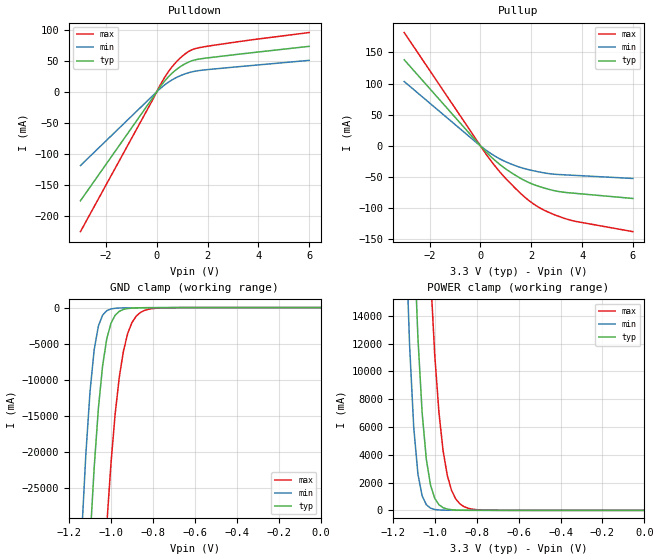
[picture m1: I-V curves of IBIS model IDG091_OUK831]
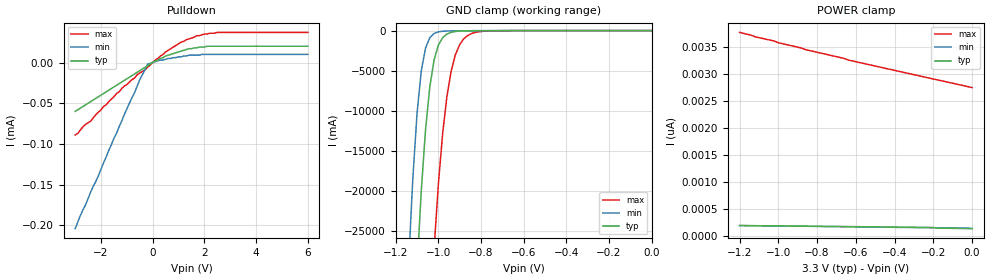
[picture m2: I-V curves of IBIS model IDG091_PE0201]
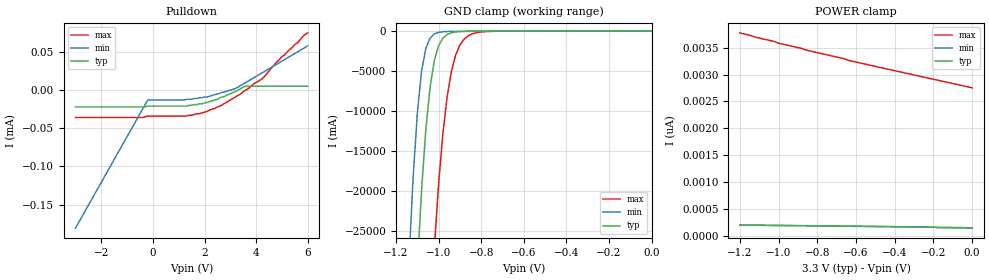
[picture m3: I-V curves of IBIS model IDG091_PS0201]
[IBIS Ver]   2.1
[File name]   dac5686.ibs
[File Rev]   1.0
[Date]   20 Oct 2004
[Source]   Preliminary Model
[Notes]
   Technology type GS30
[Disclaimer]   Please be aware that in the absence of a written agreement
|   Texas Instruments(TI) assumes no liability for:
|   (1) The accuracy of the IBIS models provided to your company
|   (2) The proper functioning of these Models in your design
|   or for any resulting applications;or
|   property rights resulting from your use of these models.
|   TI provides IBIS Models as a service to our customers and
|   therefore reserves the right to limit distribution of the
|   Models.
[Copyright]   Property of Texas Instruments Incorporated.
|   Unauthorised reproduction and/or distribution is strictly.
|   prohibited.
|   This product is protected under copyright law and trade
|   secret law as an unpublished work.
|   Created 1999,(C) Copyright 1999-2001,
|   Texas Instruments Incorporated., All Rights Reserved.
|   These commodities are under the U.S.
|   Government distribution license control.As such,they are not
|   to be re-exported without the prior approval of the U.S.
|   Department of Commerce.
[Component]   DAC5686
[Manufacturer]   Texas Instruments
[Package]
|   typ   min   max
R_pkg   0.055   0.003   0.074
L_pkg   3.746nH   2.468nH   4.445nH
C_pkg   0.413pF   0.342pF   0.498pF
[Pin]   signal_name   model_name   R_pin   L_pin   C_pin
   1   AGND   GND   0.057   4.338nH   0.438pF
   2   AVDD   POWER   0.058   4.085nH   0.472pF
   3   AVDD   POWER   0.060   4.040nH   0.456pF
   4   AGND   GND   0.060   4.008nH   0.448pF
   5   IOUTB1   NC   0.063   4.018nH   0.444pF
   6   IOUTB2   NC   0.063   3.971nH   0.427pF
   7   AGND   GND   0.063   3.935nH   0.421pF
   8   AVDD   POWER   0.064   3.883nH   0.415pF
   9   AGND   GND   0.065   3.824nH   0.403pF
   10   AVDD   POWER   0.068   3.805nH   0.392pF
   11   EXTIO   NC   0.068   3.786nH   0.384pF
   12   AGND   GND   0.069   3.777nH   0.394pF
   13   BIASJ   NC   0.067   3.733nH   0.405pF
   14   AVDD   POWER   0.069   3.778nH   0.392pF
   15   EXTLO   NC   0.065   3.785nH   0.385pF
   16   AVDD   POWER   0.065   3.827nH   0.394pF
   17   AGND   GND   0.063   3.848nH   0.403pF
   18   AVDD   POWER   0.065   3.921nH   0.416pF
   19   AGND   GND   0.062   3.955nH   0.419pF
   20   IOUTA2   NC   0.062   3.910nH   0.417pF
   21   IOUTA1   NC   0.061   3.964nH   0.439pF
   22   AGND   GND   0.060   3.962nH   0.451pF
   23   AVDD   POWER   0.057   4.045nH   0.463pF
   24   AVDD   POWER   0.003   2.474nH   0.389pF
   25   AGND   GND   0.003   2.545nH   0.342pF
   26   DVDD   POWER   0.046   3.901nH   0.416pF
   27   DGND   GND   0.046   3.704nH   0.454pF
   28   SDENB   IDG091_PE0201   0.049   3.801nH   0.445pF
   29   SCLK   IDG091_PE0201   0.049   3.745nH   0.435pF
   30   SDIO   IDG091_OUK831   0.050   3.712nH   0.426pF
   31   SDO   OUK831   0.051   3.586nH   0.402pF
   32   DVDD   POWER   0.054   3.629nH   0.402pF
   33   TXENABLE   IDG091_PE0201   0.056   3.632nH   0.401pF
   34   DA15   IDG091_PE0201   0.057   3.603nH   0.391pF
   35   DA14   IDG091_PE0201   0.057   3.584nH   0.382pF
   36   DA13   IDG091_PE0201   0.060   3.589nH   0.375pF
   37   DVDD   POWER   0.055   3.476nH   0.377pF
   38   DGND   GND   0.054   3.575nH   0.368pF
   39   DA12   IDG091_PE0201   0.052   3.487nH   0.374pF
   40   DA11   IDG091_PE0201   0.049   3.490nH   0.369pF
   41   DA10   IDG091_PE0201   0.051   3.608nH   0.383pF
   42   DA9   IDG091_PE0201   0.049   3.610nH   0.391pF
   43   DA8   IDG091_PE0201   0.049   3.739nH   0.409pF
   44   DVDD   POWER   0.050   3.767nH   0.410pF
   45   DGND   GND   0.045   3.716nH   0.410pF
   46   IOVDD   POWER   0.048   3.837nH   0.434pF
   47   IOGND   GND   0.041   3.703nH   0.440pF
   48   DA7   IDG091_PE0201   0.043   3.923nH   0.456pF
   49   DA6   IDG091_PE0201   0.003   2.468nH   0.385pF
   50   DA5   IDG091_PE0201   0.003   2.537nH   0.345pF
   51   DA4   IDG091_PE0201   0.057   4.445nH   0.457pF
   52   DA3   IDG091_PE0201   0.059   4.279nH   0.498pF
   53   DA2   IDG091_PE0201   0.062   4.315nH   0.477pF
   54   DA1   IDG091_PE0201   0.062   4.283nH   0.469pF
   55   DA0   IDG091_PE0201   0.065   4.328nH   0.468pF
   56   DVDD   POWER   0.066   4.202nH   0.444pF
   57   DGND   GND   0.066   4.126nH   0.434pF
   58   CLKGND   GND   0.065   4.106nH   0.433pF
   59   CLK1   IOH121   0.067   4.025nH   0.419pF
   60   CLK1C   IOH121   0.071   4.030nH   0.410pF
   61   CLKVDD   POWER   0.069   3.947nH   0.398pF
   62   CLK2   IOH121   0.070   3.905nH   0.405pF
   63   CLK2C   IOH121   0.073   3.898nH   0.417pF
   64   CLKGND   GND   0.074   3.911nH   0.399pF
   65   PLLGND   GND   0.073   3.916nH   0.390pF
   66   LPF   IOH121   0.073   3.956nH   0.401pF
   67   PLLVDD   POWER   0.073   3.992nH   0.410pF
   68   DVDD   POWER   0.073   4.041nH   0.421pF
   69   DGND   GND   0.070   4.042nH   0.425pF
   70   PLLLOCK   OUK831   0.069   4.043nH   0.427pF
   71   DB0   IDG091_PE0201   0.067   4.067nH   0.443pF
   72   DB1   IDG091_PE0201   0.064   4.039nH   0.448pF
   73   DB2   IDG091_PE0201   0.063   4.015nH   0.459pF
   74   DB3   IDG091_PE0201   0.060   4.174nH   0.485pF
   75   DB4   IDG091_PE0201   0.003   2.539nH   0.348pF
   76   DB5   IDG091_PE0201   0.049   3.991nH   0.426pF
   77   DB6   IDG091_PE0201   0.049   3.840nH   0.463pF
   78   DB7   IDG091_PE0201   0.050   3.788nH   0.443pF
   79   IOGND   GND   0.049   3.757nH   0.435pF
   80   IOVDD   POWER   0.051   3.777nH   0.431pF
   81   DGND   GND   0.052   3.658nH   0.407pF
   82   DVDD   POWER   0.052   3.650nH   0.403pF
   83   DB8   IDG091_PE0201   0.055   3.650nH   0.400pF
   84   DB9   IDG091_PE0201   0.055   3.597nH   0.390pF
   85   DB10   IDG091_PE0201   0.056   3.550nH   0.378pF
   86   DB11   IDG091_PE0201   0.057   3.532nH   0.370pF
   87   DB12   IDG091_PE0201   0.054   3.428nH   0.372pF
   88   DGND   GND   0.058   3.631nH   0.370pF
   89   DVDD   POWER   0.055   3.479nH   0.373pF
   90   DB13   IDG091_PE0201   0.056   3.531nH   0.369pF
   91   DB14   IDG091_PE0201   0.057   3.597nH   0.380pF
   92   DB15   IDG091_PE0201   0.056   3.611nH   0.388pF
   93   DGND   GND   0.055   3.678nH   0.403pF
   94   PHSTR   IDG091_PE0201   0.054   3.732nH   0.407pF
   95   RESETB   IDG091_PS0201   0.049   3.619nH   0.402pF
   96   SLEEP   IDG091_PE0201   0.051   3.713nH   0.425pF
   97   TESTMODE   IDG091_PE0201   0.047   3.658nH   0.433pF
   98   QFLAG   IDG091_PE0201   0.050   3.841nH   0.452pF
   99   DGND   GND   0.003   2.476nH   0.392pF
  100   DVDD   POWER   0.003   2.547nH   0.344pF
| Models and submodels in the file (5): IDG091_OUK831 (I/O), IDG091_PE0201 (Input), IDG091_PS0201 (Input), OUK831 (3-state), IOH121 (Input)
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[Model]   IDG091_OUK831
Model_type   I/O
Enable   Active-Low
Polarity   Non-Inverting
| signals   A, GZ, Y
Vinl = 0.8V
Vinh = 2.0V
Vmeas = 1.5
|   typ   min   max
C_comp   3.5921p   3.4389p   4.1227p
|   typ   min   max
[Temperature Range]   25   -40.0   125
|   typ   min   max
[Voltage Range]   3.30V   3.00V   3.60V
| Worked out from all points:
|   slope of the pulldown table from 0 to 0.495 V, typ, clamps not added: 19.3 ohm
|   slope of the pullup table from 0 to 0.495 V, typ, clamps not added: 24.2 ohm
|   GND clamp passes 1 mA (typ) near -0.58 V on its own axis
|   POWER clamp passes 1 mA (typ) near -0.64 V on its own axis
[Pulldown]
|   Voltage   I(typ)   I(min)   I(max)
-3V       -175.9mA   -119.1mA   -225.8mA
-200mV    -12.18mA   -7.956mA   -16.01mA
200mV     11.61mA    7.405mA    15.55mA
400mV     21.52mA    13.77mA    28.85mA
600mV     29.89mA    19.16mA    40.1mA
1V        42.47mA    27.25mA    57.28mA
1.3V      48.84mA    31.34mA    66.22mA
1.7V      53.08mA    34.51mA    71.52mA
3.6V      62.5mA     41.98mA    83.19mA
6V        73.47mA    50.83mA    95.74mA
[GND_clamp]
|   Voltage   I(typ)   I(min)   I(max)
-1.2V     -102.7A    -74.41A    -154.1A
-1.14V    -57.55A    -31.62A    -106.7A
-1.1V     -32.35A    -11.69A    -77.65A
-1.08V    -22.13A    -5.816A    -64.19A
-1.06V    -13.97A    -2.559A    -51.65A
-1.04V    -8.085A    -1.052A    -40.23A
-1.02V    -4.316A    -431.8mA   -30.14A
-980mV    -1.059A    -97.69mA   -14.73A
-960mV    -513.4mA   -60.94mA   -9.568A
-920mV    -131.1mA   -37.25mA   -3.566A
-880mV    -45.19mA   -28.49mA   -1.203A
0V        -130.5pA   -109.2pA   -2.072nA
[Pullup]
|   Voltage   I(typ)   I(min)   I(max)
-3V       138.1mA    103.2mA    181.7mA
-200mV    9.146mA    6.727mA    12.21mA
300mV     -12.88mA   -9.22mA    -17.63mA
900mV     -34.12mA   -23.64mA   -48.03mA
1.7V      -54.7mA    -36.06mA   -80.58mA
2.1V      -62.01mA   -39.98mA   -93.36mA
2.4V      -66.16mA   -42.43mA   -100.8mA
2.9V      -71.73mA   -45.34mA   -110.1mA
3.3V      -74.37mA   -46.38mA   -116.1mA
3.8V      -76.3mA    -47.46mA   -121.4mA
6V        -84.26mA   -52.21mA   -137.4mA
[POWER_clamp]
|   Voltage   I(typ)   I(min)   I(max)
-1.2V     83.43A     59.64A     127.8A
-1.14V    41.42A     20.8A      82.7A
-1.12V    29.85A     11.95A     68.94A
-1.1V     20.06A     5.958A     56.04A
-1.08V    12.41A     2.607A     44.19A
-1.06V    7.027A     1.048A     33.6A
-1.04V    3.679A     406.1mA    24.47A
-1.02V    1.819A     157.9mA    16.99A
-960mV    192.4mA    15.59mA    4.285A
-920mV    44.41mA    7.991mA    1.453A
-880mV    12.4mA     6.125mA    468.3mA
0V        154.5pA    161.2pA    3.029nA
[Ramp]
|   I(typ)   I(min)   I(max)
dV/dt_r   1.267/1.474n   0.957/2.769n   1.564/0.824n
dV/dt_f   1.332/1.513n   0.961/2.653n   1.616/0.826n
[Model]   IDG091_PE0201
Model_type   Input
Polarity   Non-Inverting
| signals   A, Y
Vinl = 0.8V
Vinh = 2.0V
|   typ   min   max
C_comp   3.016p   2.9215p   3.4873p
|   typ   min   max
[Temperature Range]   25   -40.0   125
|   typ   min   max
[Voltage Range]   3.30V   3.00V   3.60V
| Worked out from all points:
|   slope of the pulldown table from 0 to 0.495 V, typ, clamps not added: 62.7 kohm
|   GND clamp passes 1 mA (typ) near -0.58 V on its own axis
[Pulldown]
|   Voltage   I(typ)   I(min)   I(max)
-3V       -60uA      -204uA     -89uA
-2.6V     -52uA      -175uA     -76uA
-2.4V     -48uA      -159uA     -72uA
-2.1V     -42uA      -139uA     -61uA
-1.1V     -22uA      -64uA      -29uA
-500mV    -10uA      -21uA      -13uA
-200mV    -4uA       -2uA       -6uA
500mV     8uA        4uA        13uA
1.1V      14uA       7uA        25uA
1.7V      18uA       9uA        33uA
2.5V      20uA       10uA       37uA
6V        20uA       10uA       37uA
[GND_clamp]
|   Voltage   I(typ)   I(min)   I(max)
-1.2V     -98.78A    -71.42A    -148.8A
-1.14V    -54.21A    -29.33A    -101.8A
-1.1V     -29.69A    -10.34A    -73.18A
-1.08V    -19.94A    -5.01A     -60A
-1.06V    -12.33A    -2.162A    -47.8A
-1.04V    -6.983A    -880.6mA   -36.79A
-1.02V    -3.664A    -361.6mA   -27.18A
-980mV    -884.2mA   -83.74mA   -12.87A
-960mV    -428mA     -53.16mA   -8.232A
-920mV    -110.2mA   -33.2mA    -3A
-880mV    -38.87mA   -25.56mA   -1.002A
0V        -427.6fA   -2.728fA   -107pA
[POWER_clamp]
|   Voltage   I(typ)   I(min)   I(max)
-1.2V     197.2pA    197.2pA    3.775nA
-1.14V    194.5pA    194.5pA    3.723nA
-1.12V    194.5pA    193.6pA    3.695nA
-1.02V    191pA      190.1pA    3.613nA
-1V       191pA      189.2pA    3.583nA
-880mV    187.4pA    184.7pA    3.485nA
-860mV    187.4pA    184.7pA    3.456nA
-660mV    178.5pA    175.9pA    3.293nA
-640mV    178.1pA    175pA      3.265nA
-200mV    160.8pA    156.8pA    2.912nA
-180mV    148.8pA    155.9pA    2.896nA
0V        139.9pA    145.7pA    2.752nA
[Model]   IDG091_PS0201
Model_type   Input
Polarity   Non-Inverting
| signals   A, Y
Vinl = 0.8V
Vinh = 2.0V
|   typ   min   max
C_comp   2.9577p   2.8282p   3.4534p
|   typ   min   max
[Temperature Range]   25   -40.0   125
|   typ   min   max
[Voltage Range]   3.30V   3.00V   3.60V
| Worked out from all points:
|   GND clamp passes 1 mA (typ) near -0.58 V on its own axis
[Pulldown]
|   Voltage   I(typ)   I(min)   I(max)
-3V       -22uA      -181uA     -36uA
-400mV    -22uA      -25uA      -36uA
-200mV    -21uA      -13uA      -34uA
1.3V      -21uA      -12uA      -34uA
1.9V      -18uA      -10uA      -30uA
2.6V      -10uA      -4uA       -21uA
3.2V      -2uA       2uA        -9uA
3.6V      5uA        10uA       0A
4.3V      5uA        24uA       17uA
5V        5uA        38uA       44uA
5.8V      5uA        54uA       70uA
6V        5uA        58uA       75uA
[GND_clamp]
|   Voltage   I(typ)   I(min)   I(max)
-1.2V     -98.78A    -71.42A    -148.8A
-1.14V    -54.21A    -29.33A    -101.8A
-1.1V     -29.69A    -10.34A    -73.18A
-1.08V    -19.94A    -5.01A     -60A
-1.06V    -12.33A    -2.162A    -47.8A
-1.04V    -6.983A    -880.6mA   -36.79A
-1.02V    -3.664A    -361.6mA   -27.18A
-980mV    -884.2mA   -83.74mA   -12.87A
-960mV    -428mA     -53.16mA   -8.232A
-920mV    -110.2mA   -33.2mA    -3A
-880mV    -38.87mA   -25.56mA   -1.002A
0V        -427.6fA   -2.728fA   -107pA
[POWER_clamp]
|   Voltage   I(typ)   I(min)   I(max)
-1.2V     197.2pA    197.2pA    3.775nA
-1.14V    194.5pA    194.5pA    3.723nA
-1.12V    194.5pA    193.6pA    3.695nA
-1.02V    191pA      190.1pA    3.613nA
-1V       191pA      189.2pA    3.583nA
-880mV    187.4pA    184.7pA    3.485nA
-860mV    187.4pA    184.7pA    3.456nA
-660mV    178.5pA    175.9pA    3.293nA
-640mV    178.1pA    175pA      3.265nA
-200mV    160.8pA    156.8pA    2.912nA
-180mV    148.8pA    155.9pA    2.896nA
0V        139.9pA    145.7pA    2.752nA
